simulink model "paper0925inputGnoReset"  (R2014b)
settings: Solver=ode15s  StartTime=0.0  StopTime=24  RelTol=1e-3
libraries: fl_lib x44, nesl_utility x23, elec_lib x19, simulink x1

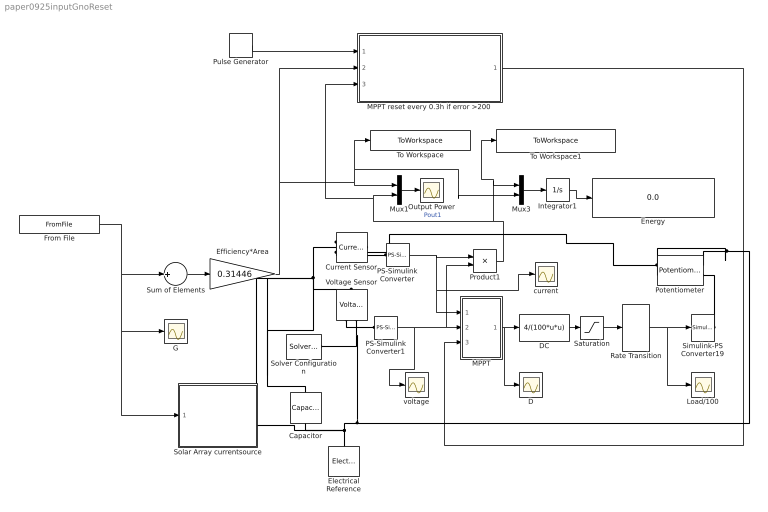
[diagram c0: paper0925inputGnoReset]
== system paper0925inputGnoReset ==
  Capacitor : fl_lib/Electrical/Electrical Elements/Capacitor  c=1e-6 F  r=1e-6 Ohm  g=0 1/Ohm  i_specify=off  i_priority=High  i=0 A  v_specify=off  v_priority=High  v=0 V  vc_specify=off  vc_priority=High  vc=0 V
  Current Sensor : fl_lib/Electrical/Electrical Sensors/Current Sensor
  D : Scope
  DC : Fcn  Expr=4/(100*u*u)
  Efficiency*Area : Gain  Gain=0.31446
  Electrical Reference : fl_lib/Electrical/Electrical Elements/Electrical Reference
  Energy : Display
  From File : FromFile  FileName=Goverlap25_4.mat  SampleTime=0
  G : Scope
  Integrator1 : Integrator
  Load/100 : Scope
  MPPT : Subsystem
  "MPPT reset every 0.3h if error >200 " : Subsystem
  Mux1 : Mux  Inputs=2
  Mux3 : Mux  Inputs=2
  Output Power : Scope
  PS-Simulink Converter : nesl_utility/PS-Simulink Converter  PhysicalDomain=network_engine_domain  SubClassName=ps_output  LeftPortType=input  RightPortType=output  PseudoPeriodic=off  Frequencies=[]  Unit=1  AffineConversion=off
  PS-Simulink Converter1 : nesl_utility/PS-Simulink Converter  PhysicalDomain=network_engine_domain  SubClassName=ps_output  LeftPortType=input  RightPortType=output  PseudoPeriodic=off  Frequencies=[]  Unit=1  AffineConversion=off
  Potentiometer : elec_lib/Passive Devices/Potentiometer  R0=100 Ohm  Rw=0.01 Ohm  Rcenter=200 Ohm  xmin=0  xmax=1  Taper=1  Gradient=1  xminL=0  xmaxL=1  lambda=1  A=1 Ohm
  Product1 : Product
  Pulse Generator : DiscretePulseGenerator  PulseType=Time based  Period=0.3  PulseWidth=0.1
  Rate Transition : RateTransition
  Saturation : Saturate  UpperLimit=1  LowerLimit=0
  Simulink-PS Converter19 : nesl_utility/Simulink-PS Converter  PhysicalDomain=network_engine_domain  SubClassName=ps_input  LeftPortType=input  RightPortType=output  PseudoPeriodic=off  Frequencies=[]  NoiseDistribution=none  NoiseParameters=[]  Unit=1  AffineConversion=off  InputFiltering=off  SimscapeFilterOrder=1  InputFilterTimeConstant=0.001  UdotUserProvided=1
  Solar Array currentsource : Subsystem
  Solver Configuration : nesl_utility/Solver Configuration  PhysicalDomain=network_engine_domain  SubClassName=solver  LeftPortType=input  RightPortType=generic  Accelerate=off  Tones=[]  Harmonics=[]  SimulateNoise=off  Profile=off  UseLocalSampling=off  EnableSwitchedLinearOptims=on  FrequencyDomain=off  UseCCode=off  RelTol=0.001  AbsTol=1e-06  MinStep=1e-09  ToWorkspace=off  DoDC=off  ResidualTolerance=1e-09  UseLocalSolver=on  LocalSolverChoice=NE_BACKWARD_EULER_ADVANCER  LocalSolverSampleTime=1e-4  DoFixedCost=on  MaxNonlinIter=3  MaxModeIter=2  LinearAlgebra=Sparse  DelaysMemoryBudget=1024  AutomaticFiltering=on  FilteringTimeConstant=0.001
  Sum of Elements : Sum  Inputs=+
  To Workspace : ToWorkspace  VariableName=Pestimated_overlap25_4  SampleTime=-1
  To Workspace1 : ToWorkspace  VariableName=Psimulated_overlap25_4  SampleTime=-1
  Voltage Sensor : fl_lib/Electrical/Electrical Sensors/Voltage Sensor
  current : Scope
  voltage : Scope
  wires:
  Sum of Elements/1 -> Efficiency*Area/1
  Product1/1 -> Mux3/1, To Workspace1/1, "MPPT reset every 0.3h if error >200 "/3(Pestimated), Mux1/2  "Pout1"
  DC/1 -> Saturation/1
  Saturation/1 -> Rate Transition/1
  MPPT/1(D) -> D/1, DC/1
  Mux1/1 -> Output Power/1
  Efficiency*Area/1 -> "MPPT reset every 0.3h if error >200 "/2(Psimulated), Mux3/2, To Workspace/1, Mux1/1
  Integrator1/1 -> Energy/1
  Mux3/1 -> Integrator1/1
  Rate Transition/1 -> Load/100/1, Simulink-PS Converter19/1
  From File/1 -> Solar Array currentsource/1(G), G/1, Sum of Elements/1
  PS-Simulink Converter1/1 -> voltage/1, Product1/2, MPPT/2(V)
  Pulse Generator/1 -> "MPPT reset every 0.3h if error >200 "/1(Check)
  PS-Simulink Converter/1 -> current/1, MPPT/1(I), Product1/1
  "MPPT reset every 0.3h if error >200 "/1(Reset Ccontrol) -> MPPT/3(Control)
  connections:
  Voltage Sensor/LConn1 -- Capacitor/LConn1 -- Solar Array currentsource/RConn1 -- Current Sensor/LConn1
  Voltage Sensor/RConn2 -- Capacitor/RConn1 -- Solar Array currentsource/RConn2 -- Potentiometer/LConn2 -- Potentiometer/RConn1 -- Electrical Reference/LConn1 -- Solver Configuration/RConn1
  Current Sensor/RConn1 -- PS-Simulink Converter/LConn1
  Voltage Sensor/RConn1 -- PS-Simulink Converter1/LConn1
  Simulink-PS Converter19/RConn1 -- Potentiometer/RConn2
  Potentiometer/LConn1 -- Current Sensor/RConn2

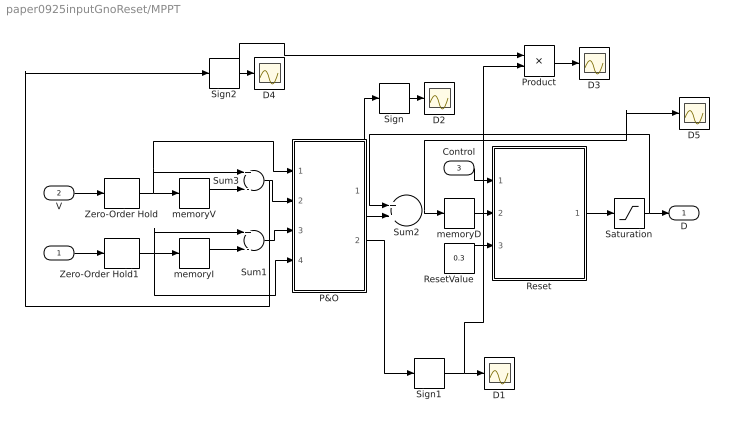
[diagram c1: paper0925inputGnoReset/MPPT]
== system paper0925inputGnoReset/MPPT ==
  I : Inport
  V : Inport  Port=2
  Control : Inport  Port=3
  D{1..5} (5 alike) : Scope
  P&O : MATLAB Function  TreatAsAtomicUnit=on
  Product : Product
  Reset : MATLAB Function  TreatAsAtomicUnit=on
  ResetValue : Constant  Value=0.3
  Saturation : Saturate  UpperLimit=1  LowerLimit=0.1
  Sign : Signum
  Sign1 : Signum
  Sign2 : Signum
  Sum1 : Sum  Inputs=+-
  Sum2 : Sum  Inputs=2
  Sum3 : Sum  Inputs=+-
  Zero-Order Hold : ZeroOrderHold  SampleTime=1e-3
  Zero-Order Hold1 : ZeroOrderHold  SampleTime=1e-3
  memoryD : Memory  X0=0.3  InheritSampleTime=on
  memoryI : Memory  InheritSampleTime=on
  memoryV : Memory  InheritSampleTime=on
  D : Outport
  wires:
  Sum2/1 -> D5/1, memoryD/1
  V/1 -> Zero-Order Hold/1
  I/1 -> Zero-Order Hold1/1
  Zero-Order Hold/1 -> P&O/1(V), Sum3/1, memoryV/1
  memoryV/1 -> Sum3/2
  Zero-Order Hold1/1 -> Sum1/1, P&O/4(I), memoryI/1
  memoryI/1 -> Sum1/2
  Saturation/1 -> Sum2/1, D/1
  Sum3/1 -> Sign2/1, P&O/2(dV)
  Sum1/1 -> P&O/3(dI)
  P&O/1(dD) -> Sum2/2, Sign/1
  ResetValue/1 -> Reset/3(ResetValue)
  memoryD/1 -> Reset/2(in)
  Reset/1(out) -> Saturation/1
  Control/1 -> Reset/1(control)
  Sign/1 -> D2/1
  Sign1/1 -> Product/2, D1/1
  P&O/2(dP) -> Sign1/1
  Product/1 -> D3/1
  Sign2/1 -> Product/1, D4/1

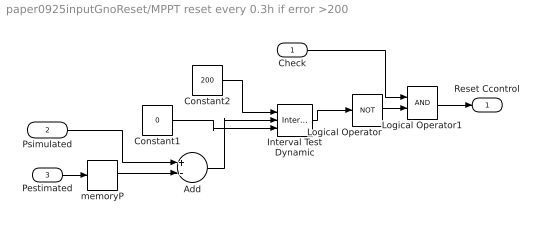
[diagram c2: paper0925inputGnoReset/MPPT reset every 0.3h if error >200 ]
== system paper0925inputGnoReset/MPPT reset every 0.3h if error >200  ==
  Check : Inport
  Psimulated : Inport  Port=2
  Pestimated : Inport  Port=3
  Add : Sum  Inputs=+-
  Constant1 : Constant  Value=0
  Constant2 : Constant  Value=200
  Interval Test Dynamic : simulink/Logic and Bit Operations/Interval Test Dynamic  IntervalClosedRight=on  IntervalClosedLeft=on  OutDataTypeStr=boolean
  Logical Operator : Logic  Operator=NOT  AllPortsSameDT=off  OutDataTypeStr=boolean
  Logical Operator1 : Logic  AllPortsSameDT=off  OutDataTypeStr=boolean
  memoryP : Memory  InheritSampleTime=on
  Reset Ccontrol : Outport
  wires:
  memoryP/1 -> Add/2
  Constant1/1 -> Interval Test Dynamic/3
  Constant2/1 -> Interval Test Dynamic/1
  Interval Test Dynamic/1 -> Logical Operator/1
  Add/1 -> Interval Test Dynamic/2
  Check/1 -> Logical Operator1/1
  Logical Operator1/1 -> Reset Ccontrol/1
  Logical Operator/1 -> Logical Operator1/2
  Pestimated/1 -> memoryP/1
  Psimulated/1 -> Add/1

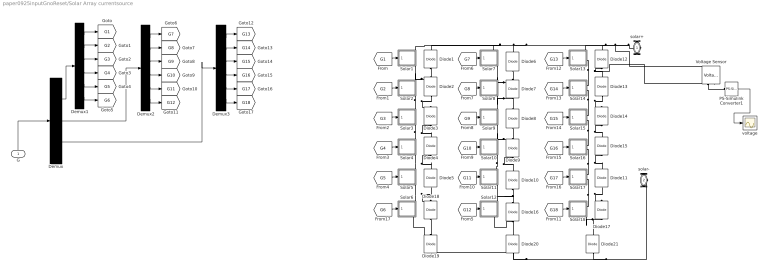
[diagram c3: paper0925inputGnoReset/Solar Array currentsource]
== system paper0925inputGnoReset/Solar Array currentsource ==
  G : Inport
  Demux : Demux  Outputs=3
  Demux1 : Demux  Outputs=6
  Demux2 : Demux  Outputs=6
  Demux3 : Demux  Outputs=6
  Diode{1..21} (21 alike) : fl_lib/Electrical/Electrical Elements/Diode  Vf=0.1 mV  Ron=0.6 Ohm  Goff=1e-10 1/Ohm  i_specify=off  i_priority=High  i=0 A  v_specify=off  v_priority=High  v=0 V
  PS-Simulink Converter1 : nesl_utility/PS-Simulink Converter  PhysicalDomain=network_engine_domain  SubClassName=ps_output  LeftPortType=input  RightPortType=output  PseudoPeriodic=off  Frequencies=[]  Unit=1  AffineConversion=off
  Solar1 : Subsystem
  Solar10 : Subsystem
  Solar11 : Subsystem
  Solar12 : Subsystem
  Solar13 : Subsystem
  Solar14 : Subsystem
  Solar15 : Subsystem
  Solar16 : Subsystem
  Solar17 : Subsystem
  Solar18 : Subsystem
  Solar2 : Subsystem
  Solar3 : Subsystem
  Solar4 : Subsystem
  Solar5 : Subsystem
  Solar6 : Subsystem
  Solar7 : Subsystem
  Solar8 : Subsystem
  Solar9 : Subsystem
  Voltage Sensor : fl_lib/Electrical/Electrical Sensors/Voltage Sensor
  voltage : Scope
  solar+ : PMIOPort  Port=1  Side=Right
  solar- : PMIOPort  Port=2  Side=Right
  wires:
  [G1] -> Solar1/1(G)
  [G2] -> Solar2/1(G)
  [G3] -> Solar3/1(G)
  G/1 -> Demux/1
  [G4] -> Solar4/1(G)
  [G7] -> Solar7/1(G)
  [G8] -> Solar8/1(G)
  [G9] -> Solar9/1(G)
  [G10] -> Solar10/1(G)
  [G11] -> Solar11/1(G)
  [G13] -> Solar13/1(G)
  [G14] -> Solar14/1(G)
  [G15] -> Solar15/1(G)
  [G16] -> Solar16/1(G)
  [G17] -> Solar17/1(G)
  Demux/1 -> Demux1/1
  Demux1/1 -> [G1]
  Demux1/2 -> [G2]
  Demux1/3 -> [G3]
  Demux1/4 -> [G4]
  Demux1/5 -> [G5]
  Demux1/6 -> [G6]
  Demux/2 -> Demux2/1
  Demux/3 -> Demux3/1
  Demux2/1 -> [G7]
  Demux2/2 -> [G8]
  Demux2/3 -> [G9]
  Demux2/4 -> [G10]
  Demux2/5 -> [G11]
  Demux2/6 -> [G12]
  Demux3/1 -> [G13]
  Demux3/2 -> [G14]
  Demux3/3 -> [G15]
  Demux3/4 -> [G16]
  Demux3/5 -> [G17]
  Demux3/6 -> [G18]
  [G6] -> Solar6/1(G)
  [G12] -> Solar12/1(G)
  [G18] -> Solar18/1(G)
  [G5] -> Solar5/1(G)
  PS-Simulink Converter1/1 -> voltage/1
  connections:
  Solar15/RConn2 -- Diode15/RConn1 -- Diode14/LConn1 -- Solar16/RConn1
  Solar13/RConn2 -- Voltage Sensor/RConn2 -- Diode13/RConn1 -- Diode12/LConn1 -- Solar14/RConn1
  Diode7/LConn1 -- Diode8/RConn1 -- Solar9/RConn1 -- Solar8/RConn2
  Solar4/RConn2 -- Diode5/RConn1 -- Diode4/LConn1 -- Solar5/RConn1
  solar+/RConn1 -- Solar1/RConn1 -- Diode1/RConn1 -- Solar7/RConn1 -- Diode6/RConn1 -- Solar13/RConn1 -- Diode12/RConn1 -- Voltage Sensor/LConn1
  Diode2/RConn1 -- Diode1/LConn1 -- Solar1/RConn2 -- Solar2/RConn1
  Diode7/RConn1 -- Diode6/LConn1 -- Solar7/RConn2 -- Solar8/RConn1
  Solar14/RConn2 -- Diode13/LConn1 -- Diode14/RConn1 -- Solar15/RConn1
  Solar2/RConn2 -- Diode2/LConn1 -- Diode3/RConn1 -- Solar3/RConn1
  Solar3/RConn2 -- Diode4/RConn1 -- Diode3/LConn1 -- Solar4/RConn1
  Diode9/RConn1 -- Diode8/LConn1 -- Solar9/RConn2 -- Solar10/RConn1
  Solar17/RConn1 -- Diode11/RConn1 -- Diode15/LConn1 -- Solar16/RConn2
  Solar10/RConn2 -- Solar11/RConn1 -- Diode10/RConn1 -- Diode9/LConn1
  Diode16/RConn1 -- Diode10/LConn1 -- Solar11/RConn2 -- Solar12/RConn1
  Solar6/RConn1 -- Diode5/LConn1 -- Diode18/RConn1 -- Solar5/RConn2
  Diode16/LConn1 -- Diode20/RConn1 -- Solar12/RConn2
  Solar18/RConn1 -- Diode11/LConn1 -- Diode17/RConn1 -- Solar17/RConn2
  Diode19/RConn1 -- Diode18/LConn1 -- Solar6/RConn2
  solar-/RConn1 -- Diode21/LConn1 -- Diode20/LConn1 -- Diode19/LConn1
  Diode17/LConn1 -- Diode21/RConn1 -- Solar18/RConn2
  Voltage Sensor/RConn1 -- PS-Simulink Converter1/LConn1

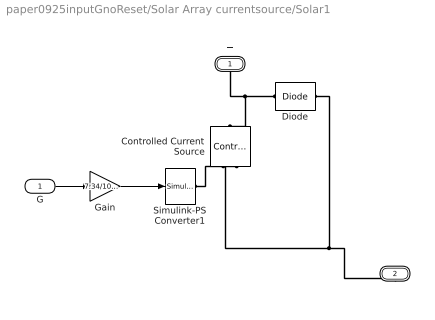
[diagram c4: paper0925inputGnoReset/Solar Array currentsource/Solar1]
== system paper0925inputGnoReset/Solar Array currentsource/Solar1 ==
  G : Inport
  Controlled Current Source : fl_lib/Electrical/Electrical Sources/Controlled Current Source
  Diode : elec_lib/Semiconductor Devices/Diode  ModelType=3  Vf=0.6 V  Ron=0.3 Ohm  Goff=1e-8 S  Rz=0.3 Ohm  Vz=50 V  C_PWL=5 pF  prmExp=2  I12=[ 0.0137 0.545 ] A  V12=[ 0.6 0.7 ] V  I1=0.0137 A  V1=0.6 V  RS=0.01 Ohm  IS=1.2614e-07 A  Tmeas=25 C  ec=117.5087  BV=Inf V  C_param=1  CJ0=5 pF  VJ=1 V  Mgrad=0.5  Vvec=[ 0.1 10 100 ] V  Cvec=[ 3.5 1 0.4 ] pF  FC=0.5  Q_param=1  Irrm=-7.15 A  iF=4 A  didt=-750 A/us  trr=115 ns  TT=50 ns  tau=100 ns  T_param=1  IS_T2=1.25e-7 A  I1_T2=0.245 A  V1_T2=0.5 V  Tmeas2=125 C  EG_param=1  EG=1.11 eV  XTI_param=1  XTI=3  dBVdT=0 V/K  Tdevice=25 C  Rth=[ 0 10 ] K/W  thermal_mass_parameterization=1  thermal_mass=[ 0 1 ] J/K  thermal_time_constant=[ 0 10 ] s  thermal_mass_initial_temperatures=[ 25 25 ] C
  Gain : Gain  Gain=7.34/1000
  Simulink-PS Converter1 : nesl_utility/Simulink-PS Converter  PhysicalDomain=network_engine_domain  SubClassName=ps_input  LeftPortType=input  RightPortType=output  PseudoPeriodic=off  Frequencies=[]  NoiseDistribution=none  NoiseParameters=[]  Unit=1  AffineConversion=off  InputFiltering=off  SimscapeFilterOrder=1  InputFilterTimeConstant=0.001  UdotUserProvided=1
  + : PMIOPort  Port=1  Side=Right
  - : PMIOPort  Port=2  Side=Right
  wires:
  G/1 -> Gain/1
  Gain/1 -> Simulink-PS Converter1/1
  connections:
  Simulink-PS Converter1/RConn1 -- Controlled Current Source/RConn1
  Diode/RConn1 -- -/RConn1 -- Controlled Current Source/RConn2
  Diode/LConn1 -- Controlled Current Source/LConn1 -- +/RConn1

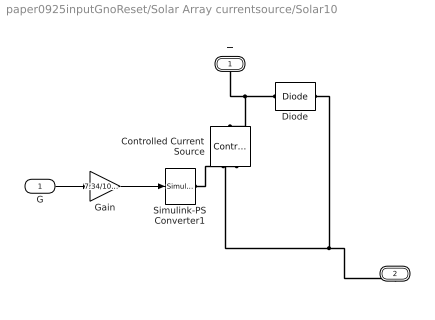
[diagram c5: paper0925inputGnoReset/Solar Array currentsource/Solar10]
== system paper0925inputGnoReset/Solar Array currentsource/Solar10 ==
  G : Inport
  Controlled Current Source : fl_lib/Electrical/Electrical Sources/Controlled Current Source
  Diode : elec_lib/Semiconductor Devices/Diode  ModelType=3  Vf=0.6 V  Ron=0.3 Ohm  Goff=1e-8 S  Rz=0.3 Ohm  Vz=50 V  C_PWL=5 pF  prmExp=2  I12=[ 0.0137 0.545 ] A  V12=[ 0.6 0.7 ] V  I1=0.0137 A  V1=0.6 V  RS=0.01 Ohm  IS=1.2614e-07 A  Tmeas=25 C  ec=117.5087  BV=Inf V  C_param=1  CJ0=5 pF  VJ=1 V  Mgrad=0.5  Vvec=[ 0.1 10 100 ] V  Cvec=[ 3.5 1 0.4 ] pF  FC=0.5  Q_param=1  Irrm=-7.15 A  iF=4 A  didt=-750 A/us  trr=115 ns  TT=50 ns  tau=100 ns  T_param=1  IS_T2=1.25e-7 A  I1_T2=0.245 A  V1_T2=0.5 V  Tmeas2=125 C  EG_param=1  EG=1.11 eV  XTI_param=1  XTI=3  dBVdT=0 V/K  Tdevice=25 C  Rth=[ 0 10 ] K/W  thermal_mass_parameterization=1  thermal_mass=[ 0 1 ] J/K  thermal_time_constant=[ 0 10 ] s  thermal_mass_initial_temperatures=[ 25 25 ] C
  Gain : Gain  Gain=7.34/1000
  Simulink-PS Converter1 : nesl_utility/Simulink-PS Converter  PhysicalDomain=network_engine_domain  SubClassName=ps_input  LeftPortType=input  RightPortType=output  PseudoPeriodic=off  Frequencies=[]  NoiseDistribution=none  NoiseParameters=[]  Unit=1  AffineConversion=off  InputFiltering=off  SimscapeFilterOrder=1  InputFilterTimeConstant=0.001  UdotUserProvided=1
  + : PMIOPort  Port=1  Side=Right
  - : PMIOPort  Port=2  Side=Right
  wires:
  G/1 -> Gain/1
  Gain/1 -> Simulink-PS Converter1/1
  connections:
  Simulink-PS Converter1/RConn1 -- Controlled Current Source/RConn1
  Diode/RConn1 -- -/RConn1 -- Controlled Current Source/RConn2
  Diode/LConn1 -- Controlled Current Source/LConn1 -- +/RConn1

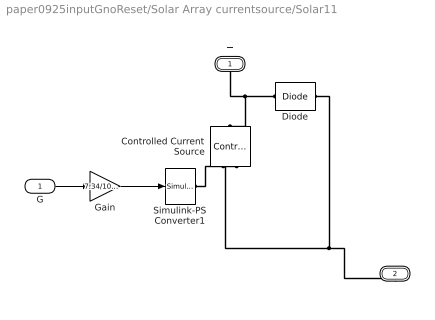
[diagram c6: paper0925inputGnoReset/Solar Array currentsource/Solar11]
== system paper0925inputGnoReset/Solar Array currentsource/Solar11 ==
  G : Inport
  Controlled Current Source : fl_lib/Electrical/Electrical Sources/Controlled Current Source
  Diode : elec_lib/Semiconductor Devices/Diode  ModelType=3  Vf=0.6 V  Ron=0.3 Ohm  Goff=1e-8 S  Rz=0.3 Ohm  Vz=50 V  C_PWL=5 pF  prmExp=2  I12=[ 0.0137 0.545 ] A  V12=[ 0.6 0.7 ] V  I1=0.0137 A  V1=0.6 V  RS=0.01 Ohm  IS=1.2614e-07 A  Tmeas=25 C  ec=117.5087  BV=Inf V  C_param=1  CJ0=5 pF  VJ=1 V  Mgrad=0.5  Vvec=[ 0.1 10 100 ] V  Cvec=[ 3.5 1 0.4 ] pF  FC=0.5  Q_param=1  Irrm=-7.15 A  iF=4 A  didt=-750 A/us  trr=115 ns  TT=50 ns  tau=100 ns  T_param=1  IS_T2=1.25e-7 A  I1_T2=0.245 A  V1_T2=0.5 V  Tmeas2=125 C  EG_param=1  EG=1.11 eV  XTI_param=1  XTI=3  dBVdT=0 V/K  Tdevice=25 C  Rth=[ 0 10 ] K/W  thermal_mass_parameterization=1  thermal_mass=[ 0 1 ] J/K  thermal_time_constant=[ 0 10 ] s  thermal_mass_initial_temperatures=[ 25 25 ] C
  Gain : Gain  Gain=7.34/1000
  Simulink-PS Converter1 : nesl_utility/Simulink-PS Converter  PhysicalDomain=network_engine_domain  SubClassName=ps_input  LeftPortType=input  RightPortType=output  PseudoPeriodic=off  Frequencies=[]  NoiseDistribution=none  NoiseParameters=[]  Unit=1  AffineConversion=off  InputFiltering=off  SimscapeFilterOrder=1  InputFilterTimeConstant=0.001  UdotUserProvided=1
  + : PMIOPort  Port=1  Side=Right
  - : PMIOPort  Port=2  Side=Right
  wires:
  G/1 -> Gain/1
  Gain/1 -> Simulink-PS Converter1/1
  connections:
  Simulink-PS Converter1/RConn1 -- Controlled Current Source/RConn1
  Diode/RConn1 -- -/RConn1 -- Controlled Current Source/RConn2
  Diode/LConn1 -- Controlled Current Source/LConn1 -- +/RConn1

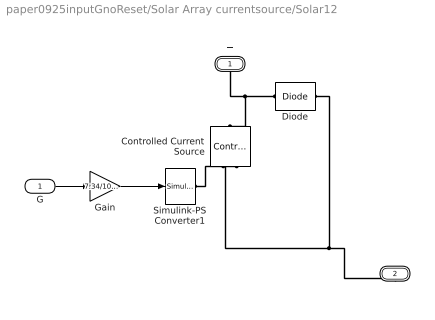
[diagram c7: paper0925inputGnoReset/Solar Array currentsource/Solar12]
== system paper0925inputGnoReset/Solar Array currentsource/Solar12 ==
  G : Inport
  Controlled Current Source : fl_lib/Electrical/Electrical Sources/Controlled Current Source
  Diode : elec_lib/Semiconductor Devices/Diode  ModelType=3  Vf=0.6 V  Ron=0.3 Ohm  Goff=1e-8 S  Rz=0.3 Ohm  Vz=50 V  C_PWL=5 pF  prmExp=2  I12=[ 0.0137 0.545 ] A  V12=[ 0.6 0.7 ] V  I1=0.0137 A  V1=0.6 V  RS=0.01 Ohm  IS=1.2614e-07 A  Tmeas=25 C  ec=117.5087  BV=Inf V  C_param=1  CJ0=5 pF  VJ=1 V  Mgrad=0.5  Vvec=[ 0.1 10 100 ] V  Cvec=[ 3.5 1 0.4 ] pF  FC=0.5  Q_param=1  Irrm=-7.15 A  iF=4 A  didt=-750 A/us  trr=115 ns  TT=50 ns  tau=100 ns  T_param=1  IS_T2=1.25e-7 A  I1_T2=0.245 A  V1_T2=0.5 V  Tmeas2=125 C  EG_param=1  EG=1.11 eV  XTI_param=1  XTI=3  dBVdT=0 V/K  Tdevice=25 C  Rth=[ 0 10 ] K/W  thermal_mass_parameterization=1  thermal_mass=[ 0 1 ] J/K  thermal_time_constant=[ 0 10 ] s  thermal_mass_initial_temperatures=[ 25 25 ] C
  Gain : Gain  Gain=7.34/1000
  Simulink-PS Converter1 : nesl_utility/Simulink-PS Converter  PhysicalDomain=network_engine_domain  SubClassName=ps_input  LeftPortType=input  RightPortType=output  PseudoPeriodic=off  Frequencies=[]  NoiseDistribution=none  NoiseParameters=[]  Unit=1  AffineConversion=off  InputFiltering=off  SimscapeFilterOrder=1  InputFilterTimeConstant=0.001  UdotUserProvided=1
  + : PMIOPort  Port=1  Side=Right
  - : PMIOPort  Port=2  Side=Right
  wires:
  G/1 -> Gain/1
  Gain/1 -> Simulink-PS Converter1/1
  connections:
  Simulink-PS Converter1/RConn1 -- Controlled Current Source/RConn1
  Diode/RConn1 -- -/RConn1 -- Controlled Current Source/RConn2
  Diode/LConn1 -- Controlled Current Source/LConn1 -- +/RConn1

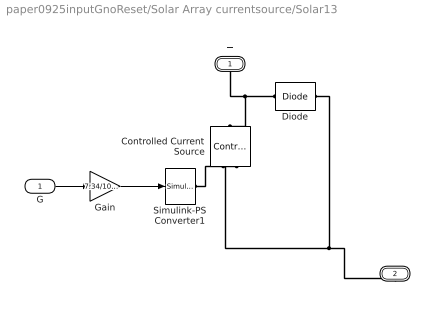
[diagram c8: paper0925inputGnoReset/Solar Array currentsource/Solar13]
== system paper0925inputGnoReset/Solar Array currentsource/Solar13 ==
  G : Inport
  Controlled Current Source : fl_lib/Electrical/Electrical Sources/Controlled Current Source
  Diode : elec_lib/Semiconductor Devices/Diode  ModelType=3  Vf=0.6 V  Ron=0.3 Ohm  Goff=1e-8 S  Rz=0.3 Ohm  Vz=50 V  C_PWL=5 pF  prmExp=2  I12=[ 0.0137 0.545 ] A  V12=[ 0.6 0.7 ] V  I1=0.0137 A  V1=0.6 V  RS=0.01 Ohm  IS=1.2614e-07 A  Tmeas=25 C  ec=117.5087  BV=Inf V  C_param=1  CJ0=5 pF  VJ=1 V  Mgrad=0.5  Vvec=[ 0.1 10 100 ] V  Cvec=[ 3.5 1 0.4 ] pF  FC=0.5  Q_param=1  Irrm=-7.15 A  iF=4 A  didt=-750 A/us  trr=115 ns  TT=50 ns  tau=100 ns  T_param=1  IS_T2=1.25e-7 A  I1_T2=0.245 A  V1_T2=0.5 V  Tmeas2=125 C  EG_param=1  EG=1.11 eV  XTI_param=1  XTI=3  dBVdT=0 V/K  Tdevice=25 C  Rth=[ 0 10 ] K/W  thermal_mass_parameterization=1  thermal_mass=[ 0 1 ] J/K  thermal_time_constant=[ 0 10 ] s  thermal_mass_initial_temperatures=[ 25 25 ] C
  Gain : Gain  Gain=7.34/1000
  Simulink-PS Converter1 : nesl_utility/Simulink-PS Converter  PhysicalDomain=network_engine_domain  SubClassName=ps_input  LeftPortType=input  RightPortType=output  PseudoPeriodic=off  Frequencies=[]  NoiseDistribution=none  NoiseParameters=[]  Unit=1  AffineConversion=off  InputFiltering=off  SimscapeFilterOrder=1  InputFilterTimeConstant=0.001  UdotUserProvided=1
  + : PMIOPort  Port=1  Side=Right
  - : PMIOPort  Port=2  Side=Right
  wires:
  G/1 -> Gain/1
  Gain/1 -> Simulink-PS Converter1/1
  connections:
  Simulink-PS Converter1/RConn1 -- Controlled Current Source/RConn1
  Diode/RConn1 -- -/RConn1 -- Controlled Current Source/RConn2
  Diode/LConn1 -- Controlled Current Source/LConn1 -- +/RConn1

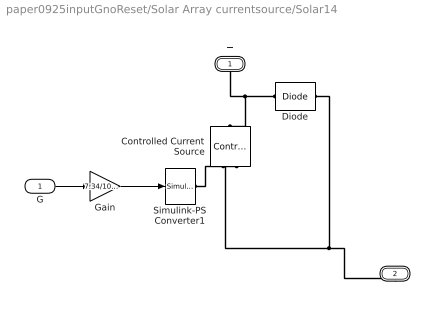
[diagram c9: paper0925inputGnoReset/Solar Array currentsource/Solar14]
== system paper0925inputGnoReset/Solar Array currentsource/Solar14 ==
  G : Inport
  Controlled Current Source : fl_lib/Electrical/Electrical Sources/Controlled Current Source
  Diode : elec_lib/Semiconductor Devices/Diode  ModelType=3  Vf=0.6 V  Ron=0.3 Ohm  Goff=1e-8 S  Rz=0.3 Ohm  Vz=50 V  C_PWL=5 pF  prmExp=2  I12=[ 0.0137 0.545 ] A  V12=[ 0.6 0.7 ] V  I1=0.0137 A  V1=0.6 V  RS=0.01 Ohm  IS=1.2614e-07 A  Tmeas=25 C  ec=117.5087  BV=Inf V  C_param=1  CJ0=5 pF  VJ=1 V  Mgrad=0.5  Vvec=[ 0.1 10 100 ] V  Cvec=[ 3.5 1 0.4 ] pF  FC=0.5  Q_param=1  Irrm=-7.15 A  iF=4 A  didt=-750 A/us  trr=115 ns  TT=50 ns  tau=100 ns  T_param=1  IS_T2=1.25e-7 A  I1_T2=0.245 A  V1_T2=0.5 V  Tmeas2=125 C  EG_param=1  EG=1.11 eV  XTI_param=1  XTI=3  dBVdT=0 V/K  Tdevice=25 C  Rth=[ 0 10 ] K/W  thermal_mass_parameterization=1  thermal_mass=[ 0 1 ] J/K  thermal_time_constant=[ 0 10 ] s  thermal_mass_initial_temperatures=[ 25 25 ] C
  Gain : Gain  Gain=7.34/1000
  Simulink-PS Converter1 : nesl_utility/Simulink-PS Converter  PhysicalDomain=network_engine_domain  SubClassName=ps_input  LeftPortType=input  RightPortType=output  PseudoPeriodic=off  Frequencies=[]  NoiseDistribution=none  NoiseParameters=[]  Unit=1  AffineConversion=off  InputFiltering=off  SimscapeFilterOrder=1  InputFilterTimeConstant=0.001  UdotUserProvided=1
  + : PMIOPort  Port=1  Side=Right
  - : PMIOPort  Port=2  Side=Right
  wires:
  G/1 -> Gain/1
  Gain/1 -> Simulink-PS Converter1/1
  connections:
  Simulink-PS Converter1/RConn1 -- Controlled Current Source/RConn1
  Diode/RConn1 -- -/RConn1 -- Controlled Current Source/RConn2
  Diode/LConn1 -- Controlled Current Source/LConn1 -- +/RConn1

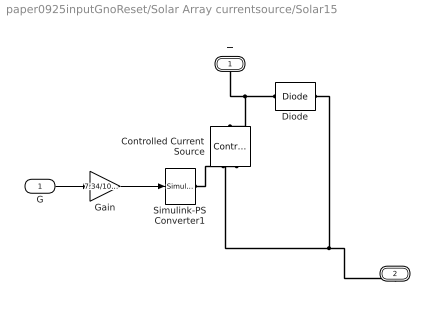
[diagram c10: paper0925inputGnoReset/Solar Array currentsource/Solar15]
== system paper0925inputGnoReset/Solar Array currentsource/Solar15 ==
  G : Inport
  Controlled Current Source : fl_lib/Electrical/Electrical Sources/Controlled Current Source
  Diode : elec_lib/Semiconductor Devices/Diode  ModelType=3  Vf=0.6 V  Ron=0.3 Ohm  Goff=1e-8 S  Rz=0.3 Ohm  Vz=50 V  C_PWL=5 pF  prmExp=2  I12=[ 0.0137 0.545 ] A  V12=[ 0.6 0.7 ] V  I1=0.0137 A  V1=0.6 V  RS=0.01 Ohm  IS=1.2614e-07 A  Tmeas=25 C  ec=117.5087  BV=Inf V  C_param=1  CJ0=5 pF  VJ=1 V  Mgrad=0.5  Vvec=[ 0.1 10 100 ] V  Cvec=[ 3.5 1 0.4 ] pF  FC=0.5  Q_param=1  Irrm=-7.15 A  iF=4 A  didt=-750 A/us  trr=115 ns  TT=50 ns  tau=100 ns  T_param=1  IS_T2=1.25e-7 A  I1_T2=0.245 A  V1_T2=0.5 V  Tmeas2=125 C  EG_param=1  EG=1.11 eV  XTI_param=1  XTI=3  dBVdT=0 V/K  Tdevice=25 C  Rth=[ 0 10 ] K/W  thermal_mass_parameterization=1  thermal_mass=[ 0 1 ] J/K  thermal_time_constant=[ 0 10 ] s  thermal_mass_initial_temperatures=[ 25 25 ] C
  Gain : Gain  Gain=7.34/1000
  Simulink-PS Converter1 : nesl_utility/Simulink-PS Converter  PhysicalDomain=network_engine_domain  SubClassName=ps_input  LeftPortType=input  RightPortType=output  PseudoPeriodic=off  Frequencies=[]  NoiseDistribution=none  NoiseParameters=[]  Unit=1  AffineConversion=off  InputFiltering=off  SimscapeFilterOrder=1  InputFilterTimeConstant=0.001  UdotUserProvided=1
  + : PMIOPort  Port=1  Side=Right
  - : PMIOPort  Port=2  Side=Right
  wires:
  G/1 -> Gain/1
  Gain/1 -> Simulink-PS Converter1/1
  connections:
  Simulink-PS Converter1/RConn1 -- Controlled Current Source/RConn1
  Diode/RConn1 -- -/RConn1 -- Controlled Current Source/RConn2
  Diode/LConn1 -- Controlled Current Source/LConn1 -- +/RConn1

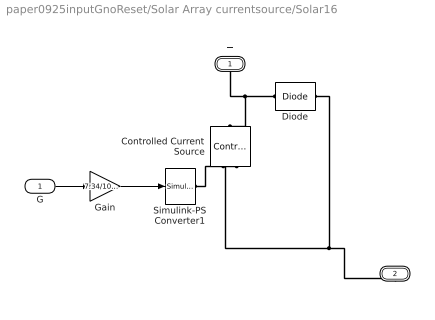
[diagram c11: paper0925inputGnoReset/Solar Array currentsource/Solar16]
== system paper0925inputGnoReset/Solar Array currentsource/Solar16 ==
  G : Inport
  Controlled Current Source : fl_lib/Electrical/Electrical Sources/Controlled Current Source
  Diode : elec_lib/Semiconductor Devices/Diode  ModelType=3  Vf=0.6 V  Ron=0.3 Ohm  Goff=1e-8 S  Rz=0.3 Ohm  Vz=50 V  C_PWL=5 pF  prmExp=2  I12=[ 0.0137 0.545 ] A  V12=[ 0.6 0.7 ] V  I1=0.0137 A  V1=0.6 V  RS=0.01 Ohm  IS=1.2614e-07 A  Tmeas=25 C  ec=117.5087  BV=Inf V  C_param=1  CJ0=5 pF  VJ=1 V  Mgrad=0.5  Vvec=[ 0.1 10 100 ] V  Cvec=[ 3.5 1 0.4 ] pF  FC=0.5  Q_param=1  Irrm=-7.15 A  iF=4 A  didt=-750 A/us  trr=115 ns  TT=50 ns  tau=100 ns  T_param=1  IS_T2=1.25e-7 A  I1_T2=0.245 A  V1_T2=0.5 V  Tmeas2=125 C  EG_param=1  EG=1.11 eV  XTI_param=1  XTI=3  dBVdT=0 V/K  Tdevice=25 C  Rth=[ 0 10 ] K/W  thermal_mass_parameterization=1  thermal_mass=[ 0 1 ] J/K  thermal_time_constant=[ 0 10 ] s  thermal_mass_initial_temperatures=[ 25 25 ] C
  Gain : Gain  Gain=7.34/1000
  Simulink-PS Converter1 : nesl_utility/Simulink-PS Converter  PhysicalDomain=network_engine_domain  SubClassName=ps_input  LeftPortType=input  RightPortType=output  PseudoPeriodic=off  Frequencies=[]  NoiseDistribution=none  NoiseParameters=[]  Unit=1  AffineConversion=off  InputFiltering=off  SimscapeFilterOrder=1  InputFilterTimeConstant=0.001  UdotUserProvided=1
  + : PMIOPort  Port=1  Side=Right
  - : PMIOPort  Port=2  Side=Right
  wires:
  G/1 -> Gain/1
  Gain/1 -> Simulink-PS Converter1/1
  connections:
  Simulink-PS Converter1/RConn1 -- Controlled Current Source/RConn1
  Diode/RConn1 -- -/RConn1 -- Controlled Current Source/RConn2
  Diode/LConn1 -- Controlled Current Source/LConn1 -- +/RConn1

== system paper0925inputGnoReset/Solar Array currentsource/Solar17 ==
  G : Inport
  Controlled Current Source : fl_lib/Electrical/Electrical Sources/Controlled Current Source
  Diode : elec_lib/Semiconductor Devices/Diode  ModelType=3  Vf=0.6 V  Ron=0.3 Ohm  Goff=1e-8 S  Rz=0.3 Ohm  Vz=50 V  C_PWL=5 pF  prmExp=2  I12=[ 0.0137 0.545 ] A  V12=[ 0.6 0.7 ] V  I1=0.0137 A  V1=0.6 V  RS=0.01 Ohm  IS=1.2614e-07 A  Tmeas=25 C  ec=117.5087  BV=Inf V  C_param=1  CJ0=5 pF  VJ=1 V  Mgrad=0.5  Vvec=[ 0.1 10 100 ] V  Cvec=[ 3.5 1 0.4 ] pF  FC=0.5  Q_param=1  Irrm=-7.15 A  iF=4 A  didt=-750 A/us  trr=115 ns  TT=50 ns  tau=100 ns  T_param=1  IS_T2=1.25e-7 A  I1_T2=0.245 A  V1_T2=0.5 V  Tmeas2=125 C  EG_param=1  EG=1.11 eV  XTI_param=1  XTI=3  dBVdT=0 V/K  Tdevice=25 C  Rth=[ 0 10 ] K/W  thermal_mass_parameterization=1  thermal_mass=[ 0 1 ] J/K  thermal_time_constant=[ 0 10 ] s  thermal_mass_initial_temperatures=[ 25 25 ] C
  Gain : Gain  Gain=7.34/1000
  Simulink-PS Converter1 : nesl_utility/Simulink-PS Converter  PhysicalDomain=network_engine_domain  SubClassName=ps_input  LeftPortType=input  RightPortType=output  PseudoPeriodic=off  Frequencies=[]  NoiseDistribution=none  NoiseParameters=[]  Unit=1  AffineConversion=off  InputFiltering=off  SimscapeFilterOrder=1  InputFilterTimeConstant=0.001  UdotUserProvided=1
  + : PMIOPort  Port=1  Side=Right
  - : PMIOPort  Port=2  Side=Right
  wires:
  G/1 -> Gain/1
  Gain/1 -> Simulink-PS Converter1/1
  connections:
  Simulink-PS Converter1/RConn1 -- Controlled Current Source/RConn1
  Diode/RConn1 -- -/RConn1 -- Controlled Current Source/RConn2
  Diode/LConn1 -- Controlled Current Source/LConn1 -- +/RConn1

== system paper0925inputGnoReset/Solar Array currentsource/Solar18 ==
  G : Inport
  Controlled Current Source : fl_lib/Electrical/Electrical Sources/Controlled Current Source
  Diode : elec_lib/Semiconductor Devices/Diode  ModelType=3  Vf=0.6 V  Ron=0.3 Ohm  Goff=1e-8 S  Rz=0.3 Ohm  Vz=50 V  C_PWL=5 pF  prmExp=2  I12=[ 0.0137 0.545 ] A  V12=[ 0.6 0.7 ] V  I1=0.0137 A  V1=0.6 V  RS=0.01 Ohm  IS=1.2614e-07 A  Tmeas=25 C  ec=117.5087  BV=Inf V  C_param=1  CJ0=5 pF  VJ=1 V  Mgrad=0.5  Vvec=[ 0.1 10 100 ] V  Cvec=[ 3.5 1 0.4 ] pF  FC=0.5  Q_param=1  Irrm=-7.15 A  iF=4 A  didt=-750 A/us  trr=115 ns  TT=50 ns  tau=100 ns  T_param=1  IS_T2=1.25e-7 A  I1_T2=0.245 A  V1_T2=0.5 V  Tmeas2=125 C  EG_param=1  EG=1.11 eV  XTI_param=1  XTI=3  dBVdT=0 V/K  Tdevice=25 C  Rth=[ 0 10 ] K/W  thermal_mass_parameterization=1  thermal_mass=[ 0 1 ] J/K  thermal_time_constant=[ 0 10 ] s  thermal_mass_initial_temperatures=[ 25 25 ] C
  Gain : Gain  Gain=7.34/1000
  Simulink-PS Converter1 : nesl_utility/Simulink-PS Converter  PhysicalDomain=network_engine_domain  SubClassName=ps_input  LeftPortType=input  RightPortType=output  PseudoPeriodic=off  Frequencies=[]  NoiseDistribution=none  NoiseParameters=[]  Unit=1  AffineConversion=off  InputFiltering=off  SimscapeFilterOrder=1  InputFilterTimeConstant=0.001  UdotUserProvided=1
  + : PMIOPort  Port=1  Side=Right
  - : PMIOPort  Port=2  Side=Right
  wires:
  G/1 -> Gain/1
  Gain/1 -> Simulink-PS Converter1/1
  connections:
  Simulink-PS Converter1/RConn1 -- Controlled Current Source/RConn1
  Diode/RConn1 -- -/RConn1 -- Controlled Current Source/RConn2
  Diode/LConn1 -- Controlled Current Source/LConn1 -- +/RConn1

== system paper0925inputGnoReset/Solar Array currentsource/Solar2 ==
  G : Inport
  Controlled Current Source : fl_lib/Electrical/Electrical Sources/Controlled Current Source
  Diode : elec_lib/Semiconductor Devices/Diode  ModelType=3  Vf=0.6 V  Ron=0.3 Ohm  Goff=1e-8 S  Rz=0.3 Ohm  Vz=50 V  C_PWL=5 pF  prmExp=2  I12=[ 0.0137 0.545 ] A  V12=[ 0.6 0.7 ] V  I1=0.0137 A  V1=0.6 V  RS=0.01 Ohm  IS=1.2614e-07 A  Tmeas=25 C  ec=117.5087  BV=Inf V  C_param=1  CJ0=5 pF  VJ=1 V  Mgrad=0.5  Vvec=[ 0.1 10 100 ] V  Cvec=[ 3.5 1 0.4 ] pF  FC=0.5  Q_param=1  Irrm=-7.15 A  iF=4 A  didt=-750 A/us  trr=115 ns  TT=50 ns  tau=100 ns  T_param=1  IS_T2=1.25e-7 A  I1_T2=0.245 A  V1_T2=0.5 V  Tmeas2=125 C  EG_param=1  EG=1.11 eV  XTI_param=1  XTI=3  dBVdT=0 V/K  Tdevice=25 C  Rth=[ 0 10 ] K/W  thermal_mass_parameterization=1  thermal_mass=[ 0 1 ] J/K  thermal_time_constant=[ 0 10 ] s  thermal_mass_initial_temperatures=[ 25 25 ] C
  Gain : Gain  Gain=7.34/1000
  Simulink-PS Converter1 : nesl_utility/Simulink-PS Converter  PhysicalDomain=network_engine_domain  SubClassName=ps_input  LeftPortType=input  RightPortType=output  PseudoPeriodic=off  Frequencies=[]  NoiseDistribution=none  NoiseParameters=[]  Unit=1  AffineConversion=off  InputFiltering=off  SimscapeFilterOrder=1  InputFilterTimeConstant=0.001  UdotUserProvided=1
  + : PMIOPort  Port=1  Side=Right
  - : PMIOPort  Port=2  Side=Right
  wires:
  G/1 -> Gain/1
  Gain/1 -> Simulink-PS Converter1/1
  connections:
  Simulink-PS Converter1/RConn1 -- Controlled Current Source/RConn1
  Diode/RConn1 -- -/RConn1 -- Controlled Current Source/RConn2
  Diode/LConn1 -- Controlled Current Source/LConn1 -- +/RConn1

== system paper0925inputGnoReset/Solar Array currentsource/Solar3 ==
  G : Inport
  Controlled Current Source : fl_lib/Electrical/Electrical Sources/Controlled Current Source
  Diode : elec_lib/Semiconductor Devices/Diode  ModelType=3  Vf=0.6 V  Ron=0.3 Ohm  Goff=1e-8 S  Rz=0.3 Ohm  Vz=50 V  C_PWL=5 pF  prmExp=2  I12=[ 0.0137 0.545 ] A  V12=[ 0.6 0.7 ] V  I1=0.0137 A  V1=0.6 V  RS=0.01 Ohm  IS=1.2614e-07 A  Tmeas=25 C  ec=117.5087  BV=Inf V  C_param=1  CJ0=5 pF  VJ=1 V  Mgrad=0.5  Vvec=[ 0.1 10 100 ] V  Cvec=[ 3.5 1 0.4 ] pF  FC=0.5  Q_param=1  Irrm=-7.15 A  iF=4 A  didt=-750 A/us  trr=115 ns  TT=50 ns  tau=100 ns  T_param=1  IS_T2=1.25e-7 A  I1_T2=0.245 A  V1_T2=0.5 V  Tmeas2=125 C  EG_param=1  EG=1.11 eV  XTI_param=1  XTI=3  dBVdT=0 V/K  Tdevice=25 C  Rth=[ 0 10 ] K/W  thermal_mass_parameterization=1  thermal_mass=[ 0 1 ] J/K  thermal_time_constant=[ 0 10 ] s  thermal_mass_initial_temperatures=[ 25 25 ] C
  Gain : Gain  Gain=7.34/1000
  Simulink-PS Converter1 : nesl_utility/Simulink-PS Converter  PhysicalDomain=network_engine_domain  SubClassName=ps_input  LeftPortType=input  RightPortType=output  PseudoPeriodic=off  Frequencies=[]  NoiseDistribution=none  NoiseParameters=[]  Unit=1  AffineConversion=off  InputFiltering=off  SimscapeFilterOrder=1  InputFilterTimeConstant=0.001  UdotUserProvided=1
  + : PMIOPort  Port=1  Side=Right
  - : PMIOPort  Port=2  Side=Right
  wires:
  G/1 -> Gain/1
  Gain/1 -> Simulink-PS Converter1/1
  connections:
  Simulink-PS Converter1/RConn1 -- Controlled Current Source/RConn1
  Diode/RConn1 -- -/RConn1 -- Controlled Current Source/RConn2
  Diode/LConn1 -- Controlled Current Source/LConn1 -- +/RConn1

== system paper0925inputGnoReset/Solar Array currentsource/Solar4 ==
  G : Inport
  Controlled Current Source : fl_lib/Electrical/Electrical Sources/Controlled Current Source
  Diode : elec_lib/Semiconductor Devices/Diode  ModelType=3  Vf=0.6 V  Ron=0.3 Ohm  Goff=1e-8 S  Rz=0.3 Ohm  Vz=50 V  C_PWL=5 pF  prmExp=2  I12=[ 0.0137 0.545 ] A  V12=[ 0.6 0.7 ] V  I1=0.0137 A  V1=0.6 V  RS=0.01 Ohm  IS=1.2614e-07 A  Tmeas=25 C  ec=117.5087  BV=Inf V  C_param=1  CJ0=5 pF  VJ=1 V  Mgrad=0.5  Vvec=[ 0.1 10 100 ] V  Cvec=[ 3.5 1 0.4 ] pF  FC=0.5  Q_param=1  Irrm=-7.15 A  iF=4 A  didt=-750 A/us  trr=115 ns  TT=50 ns  tau=100 ns  T_param=1  IS_T2=1.25e-7 A  I1_T2=0.245 A  V1_T2=0.5 V  Tmeas2=125 C  EG_param=1  EG=1.11 eV  XTI_param=1  XTI=3  dBVdT=0 V/K  Tdevice=25 C  Rth=[ 0 10 ] K/W  thermal_mass_parameterization=1  thermal_mass=[ 0 1 ] J/K  thermal_time_constant=[ 0 10 ] s  thermal_mass_initial_temperatures=[ 25 25 ] C
  Gain : Gain  Gain=7.34/1000
  Simulink-PS Converter1 : nesl_utility/Simulink-PS Converter  PhysicalDomain=network_engine_domain  SubClassName=ps_input  LeftPortType=input  RightPortType=output  PseudoPeriodic=off  Frequencies=[]  NoiseDistribution=none  NoiseParameters=[]  Unit=1  AffineConversion=off  InputFiltering=off  SimscapeFilterOrder=1  InputFilterTimeConstant=0.001  UdotUserProvided=1
  + : PMIOPort  Port=1  Side=Right
  - : PMIOPort  Port=2  Side=Right
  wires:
  G/1 -> Gain/1
  Gain/1 -> Simulink-PS Converter1/1
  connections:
  Simulink-PS Converter1/RConn1 -- Controlled Current Source/RConn1
  Diode/RConn1 -- -/RConn1 -- Controlled Current Source/RConn2
  Diode/LConn1 -- Controlled Current Source/LConn1 -- +/RConn1

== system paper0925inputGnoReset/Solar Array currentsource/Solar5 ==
  G : Inport
  Controlled Current Source : fl_lib/Electrical/Electrical Sources/Controlled Current Source
  Diode : elec_lib/Semiconductor Devices/Diode  ModelType=3  Vf=0.6 V  Ron=0.3 Ohm  Goff=1e-8 S  Rz=0.3 Ohm  Vz=50 V  C_PWL=5 pF  prmExp=2  I12=[ 0.0137 0.545 ] A  V12=[ 0.6 0.7 ] V  I1=0.0137 A  V1=0.6 V  RS=0.01 Ohm  IS=1.2614e-07 A  Tmeas=25 C  ec=117.5087  BV=Inf V  C_param=1  CJ0=5 pF  VJ=1 V  Mgrad=0.5  Vvec=[ 0.1 10 100 ] V  Cvec=[ 3.5 1 0.4 ] pF  FC=0.5  Q_param=1  Irrm=-7.15 A  iF=4 A  didt=-750 A/us  trr=115 ns  TT=50 ns  tau=100 ns  T_param=1  IS_T2=1.25e-7 A  I1_T2=0.245 A  V1_T2=0.5 V  Tmeas2=125 C  EG_param=1  EG=1.11 eV  XTI_param=1  XTI=3  dBVdT=0 V/K  Tdevice=25 C  Rth=[ 0 10 ] K/W  thermal_mass_parameterization=1  thermal_mass=[ 0 1 ] J/K  thermal_time_constant=[ 0 10 ] s  thermal_mass_initial_temperatures=[ 25 25 ] C
  Gain : Gain  Gain=7.34/1000
  Simulink-PS Converter1 : nesl_utility/Simulink-PS Converter  PhysicalDomain=network_engine_domain  SubClassName=ps_input  LeftPortType=input  RightPortType=output  PseudoPeriodic=off  Frequencies=[]  NoiseDistribution=none  NoiseParameters=[]  Unit=1  AffineConversion=off  InputFiltering=off  SimscapeFilterOrder=1  InputFilterTimeConstant=0.001  UdotUserProvided=1
  + : PMIOPort  Port=1  Side=Right
  - : PMIOPort  Port=2  Side=Right
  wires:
  G/1 -> Gain/1
  Gain/1 -> Simulink-PS Converter1/1
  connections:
  Simulink-PS Converter1/RConn1 -- Controlled Current Source/RConn1
  Diode/RConn1 -- -/RConn1 -- Controlled Current Source/RConn2
  Diode/LConn1 -- Controlled Current Source/LConn1 -- +/RConn1

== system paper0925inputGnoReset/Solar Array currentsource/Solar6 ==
  G : Inport
  Controlled Current Source : fl_lib/Electrical/Electrical Sources/Controlled Current Source
  Diode : elec_lib/Semiconductor Devices/Diode  ModelType=3  Vf=0.6 V  Ron=0.3 Ohm  Goff=1e-8 S  Rz=0.3 Ohm  Vz=50 V  C_PWL=5 pF  prmExp=2  I12=[ 0.0137 0.545 ] A  V12=[ 0.6 0.7 ] V  I1=0.0137 A  V1=0.6 V  RS=0.01 Ohm  IS=1.2614e-07 A  Tmeas=25 C  ec=117.5087  BV=Inf V  C_param=1  CJ0=5 pF  VJ=1 V  Mgrad=0.5  Vvec=[ 0.1 10 100 ] V  Cvec=[ 3.5 1 0.4 ] pF  FC=0.5  Q_param=1  Irrm=-7.15 A  iF=4 A  didt=-750 A/us  trr=115 ns  TT=50 ns  tau=100 ns  T_param=1  IS_T2=1.25e-7 A  I1_T2=0.245 A  V1_T2=0.5 V  Tmeas2=125 C  EG_param=1  EG=1.11 eV  XTI_param=1  XTI=3  dBVdT=0 V/K  Tdevice=25 C  Rth=[ 0 10 ] K/W  thermal_mass_parameterization=1  thermal_mass=[ 0 1 ] J/K  thermal_time_constant=[ 0 10 ] s  thermal_mass_initial_temperatures=[ 25 25 ] C
  Gain : Gain  Gain=7.34/1000
  Simulink-PS Converter1 : nesl_utility/Simulink-PS Converter  PhysicalDomain=network_engine_domain  SubClassName=ps_input  LeftPortType=input  RightPortType=output  PseudoPeriodic=off  Frequencies=[]  NoiseDistribution=none  NoiseParameters=[]  Unit=1  AffineConversion=off  InputFiltering=off  SimscapeFilterOrder=1  InputFilterTimeConstant=0.001  UdotUserProvided=1
  + : PMIOPort  Port=1  Side=Right
  - : PMIOPort  Port=2  Side=Right
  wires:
  G/1 -> Gain/1
  Gain/1 -> Simulink-PS Converter1/1
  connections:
  Simulink-PS Converter1/RConn1 -- Controlled Current Source/RConn1
  Diode/RConn1 -- -/RConn1 -- Controlled Current Source/RConn2
  Diode/LConn1 -- Controlled Current Source/LConn1 -- +/RConn1

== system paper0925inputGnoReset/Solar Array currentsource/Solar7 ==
  G : Inport
  Controlled Current Source : fl_lib/Electrical/Electrical Sources/Controlled Current Source
  Diode : elec_lib/Semiconductor Devices/Diode  ModelType=3  Vf=0.6 V  Ron=0.3 Ohm  Goff=1e-8 S  Rz=0.3 Ohm  Vz=50 V  C_PWL=5 pF  prmExp=2  I12=[ 0.0137 0.545 ] A  V12=[ 0.6 0.7 ] V  I1=0.0137 A  V1=0.6 V  RS=0.01 Ohm  IS=1.2614e-07 A  Tmeas=25 C  ec=117.5087  BV=Inf V  C_param=1  CJ0=5 pF  VJ=1 V  Mgrad=0.5  Vvec=[ 0.1 10 100 ] V  Cvec=[ 3.5 1 0.4 ] pF  FC=0.5  Q_param=1  Irrm=-7.15 A  iF=4 A  didt=-750 A/us  trr=115 ns  TT=50 ns  tau=100 ns  T_param=1  IS_T2=1.25e-7 A  I1_T2=0.245 A  V1_T2=0.5 V  Tmeas2=125 C  EG_param=1  EG=1.11 eV  XTI_param=1  XTI=3  dBVdT=0 V/K  Tdevice=25 C  Rth=[ 0 10 ] K/W  thermal_mass_parameterization=1  thermal_mass=[ 0 1 ] J/K  thermal_time_constant=[ 0 10 ] s  thermal_mass_initial_temperatures=[ 25 25 ] C
  Gain : Gain  Gain=7.34/1000
  Simulink-PS Converter1 : nesl_utility/Simulink-PS Converter  PhysicalDomain=network_engine_domain  SubClassName=ps_input  LeftPortType=input  RightPortType=output  PseudoPeriodic=off  Frequencies=[]  NoiseDistribution=none  NoiseParameters=[]  Unit=1  AffineConversion=off  InputFiltering=off  SimscapeFilterOrder=1  InputFilterTimeConstant=0.001  UdotUserProvided=1
  + : PMIOPort  Port=1  Side=Right
  - : PMIOPort  Port=2  Side=Right
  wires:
  G/1 -> Gain/1
  Gain/1 -> Simulink-PS Converter1/1
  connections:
  Simulink-PS Converter1/RConn1 -- Controlled Current Source/RConn1
  Diode/RConn1 -- -/RConn1 -- Controlled Current Source/RConn2
  Diode/LConn1 -- Controlled Current Source/LConn1 -- +/RConn1

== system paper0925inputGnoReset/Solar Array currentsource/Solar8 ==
  G : Inport
  Controlled Current Source : fl_lib/Electrical/Electrical Sources/Controlled Current Source
  Diode : elec_lib/Semiconductor Devices/Diode  ModelType=3  Vf=0.6 V  Ron=0.3 Ohm  Goff=1e-8 S  Rz=0.3 Ohm  Vz=50 V  C_PWL=5 pF  prmExp=2  I12=[ 0.0137 0.545 ] A  V12=[ 0.6 0.7 ] V  I1=0.0137 A  V1=0.6 V  RS=0.01 Ohm  IS=1.2614e-07 A  Tmeas=25 C  ec=117.5087  BV=Inf V  C_param=1  CJ0=5 pF  VJ=1 V  Mgrad=0.5  Vvec=[ 0.1 10 100 ] V  Cvec=[ 3.5 1 0.4 ] pF  FC=0.5  Q_param=1  Irrm=-7.15 A  iF=4 A  didt=-750 A/us  trr=115 ns  TT=50 ns  tau=100 ns  T_param=1  IS_T2=1.25e-7 A  I1_T2=0.245 A  V1_T2=0.5 V  Tmeas2=125 C  EG_param=1  EG=1.11 eV  XTI_param=1  XTI=3  dBVdT=0 V/K  Tdevice=25 C  Rth=[ 0 10 ] K/W  thermal_mass_parameterization=1  thermal_mass=[ 0 1 ] J/K  thermal_time_constant=[ 0 10 ] s  thermal_mass_initial_temperatures=[ 25 25 ] C
  Gain : Gain  Gain=7.34/1000
  Simulink-PS Converter1 : nesl_utility/Simulink-PS Converter  PhysicalDomain=network_engine_domain  SubClassName=ps_input  LeftPortType=input  RightPortType=output  PseudoPeriodic=off  Frequencies=[]  NoiseDistribution=none  NoiseParameters=[]  Unit=1  AffineConversion=off  InputFiltering=off  SimscapeFilterOrder=1  InputFilterTimeConstant=0.001  UdotUserProvided=1
  + : PMIOPort  Port=1  Side=Right
  - : PMIOPort  Port=2  Side=Right
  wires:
  G/1 -> Gain/1
  Gain/1 -> Simulink-PS Converter1/1
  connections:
  Simulink-PS Converter1/RConn1 -- Controlled Current Source/RConn1
  Diode/RConn1 -- -/RConn1 -- Controlled Current Source/RConn2
  Diode/LConn1 -- Controlled Current Source/LConn1 -- +/RConn1

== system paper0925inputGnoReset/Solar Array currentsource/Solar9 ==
  G : Inport
  Controlled Current Source : fl_lib/Electrical/Electrical Sources/Controlled Current Source
  Diode : elec_lib/Semiconductor Devices/Diode  ModelType=3  Vf=0.6 V  Ron=0.3 Ohm  Goff=1e-8 S  Rz=0.3 Ohm  Vz=50 V  C_PWL=5 pF  prmExp=2  I12=[ 0.0137 0.545 ] A  V12=[ 0.6 0.7 ] V  I1=0.0137 A  V1=0.6 V  RS=0.01 Ohm  IS=1.2614e-07 A  Tmeas=25 C  ec=117.5087  BV=Inf V  C_param=1  CJ0=5 pF  VJ=1 V  Mgrad=0.5  Vvec=[ 0.1 10 100 ] V  Cvec=[ 3.5 1 0.4 ] pF  FC=0.5  Q_param=1  Irrm=-7.15 A  iF=4 A  didt=-750 A/us  trr=115 ns  TT=50 ns  tau=100 ns  T_param=1  IS_T2=1.25e-7 A  I1_T2=0.245 A  V1_T2=0.5 V  Tmeas2=125 C  EG_param=1  EG=1.11 eV  XTI_param=1  XTI=3  dBVdT=0 V/K  Tdevice=25 C  Rth=[ 0 10 ] K/W  thermal_mass_parameterization=1  thermal_mass=[ 0 1 ] J/K  thermal_time_constant=[ 0 10 ] s  thermal_mass_initial_temperatures=[ 25 25 ] C
  Gain : Gain  Gain=7.34/1000
  Simulink-PS Converter1 : nesl_utility/Simulink-PS Converter  PhysicalDomain=network_engine_domain  SubClassName=ps_input  LeftPortType=input  RightPortType=output  PseudoPeriodic=off  Frequencies=[]  NoiseDistribution=none  NoiseParameters=[]  Unit=1  AffineConversion=off  InputFiltering=off  SimscapeFilterOrder=1  InputFilterTimeConstant=0.001  UdotUserProvided=1
  + : PMIOPort  Port=1  Side=Right
  - : PMIOPort  Port=2  Side=Right
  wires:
  G/1 -> Gain/1
  Gain/1 -> Simulink-PS Converter1/1
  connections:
  Simulink-PS Converter1/RConn1 -- Controlled Current Source/RConn1
  Diode/RConn1 -- -/RConn1 -- Controlled Current Source/RConn2
  Diode/LConn1 -- Controlled Current Source/LConn1 -- +/RConn1

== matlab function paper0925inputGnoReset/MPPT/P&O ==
function [dD,dP]  = fcn(V,dV,dI,I)
%#codegen
step=0.001;

dP=(V+dV).*(I+dI)-V.*I;
% dD=-1*sign(dP)*sign(dV)*step;
if abs(dP) > 1e-6
    if dP < 0
        if dV < 0
            dD = -step;
        else
            dD = step;
        end
    else
        if dV < 0
            dD = step;
        else
            dD = -step;
        end
    end
else dD=0;
end

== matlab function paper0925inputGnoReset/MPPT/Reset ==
function out  = fcn(control,in,ResetValue)
%#codegen

if control ==1
    out=ResetValue;
else
    out=in;
end
